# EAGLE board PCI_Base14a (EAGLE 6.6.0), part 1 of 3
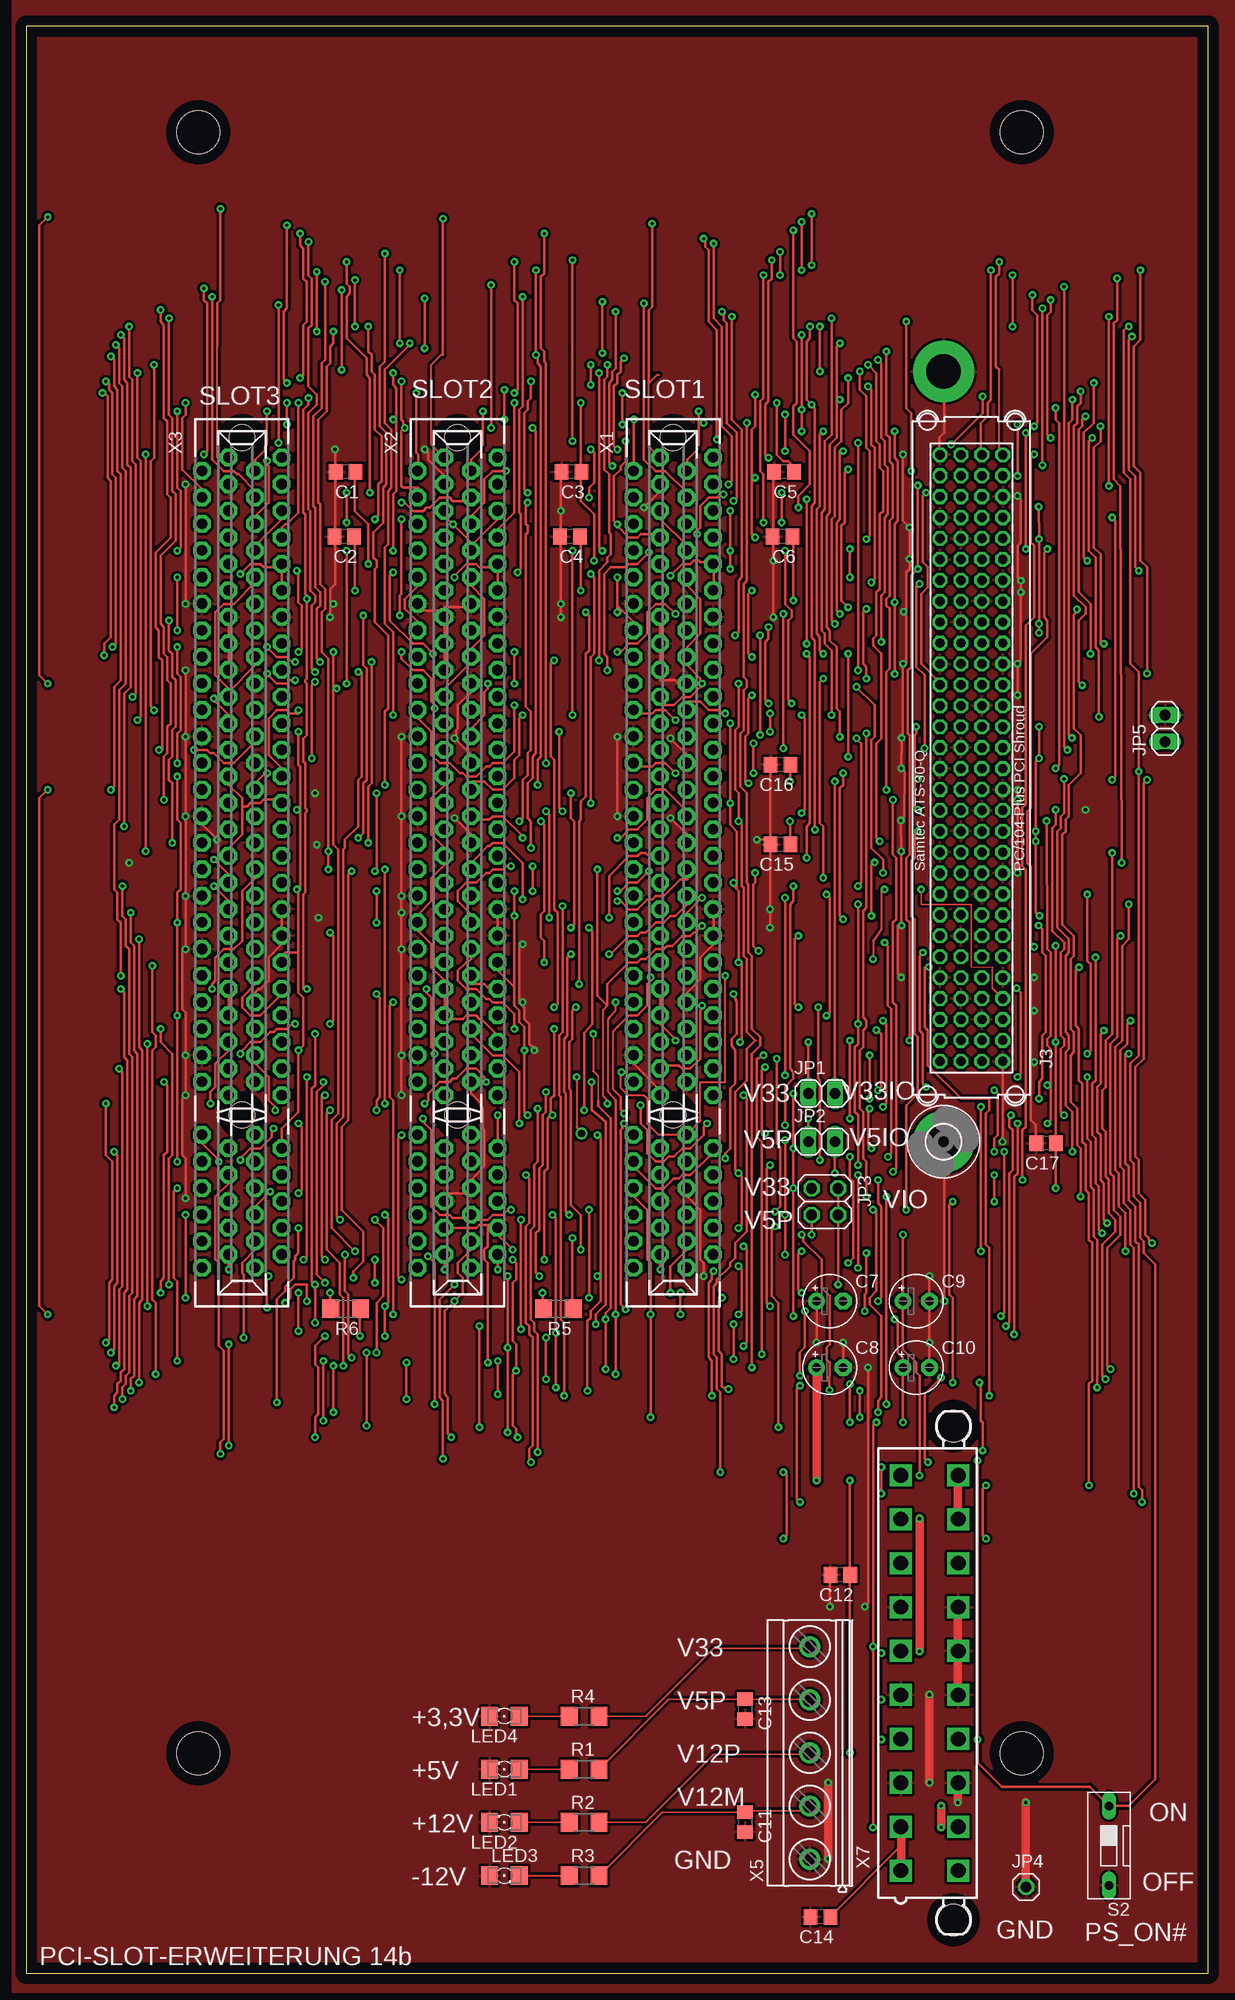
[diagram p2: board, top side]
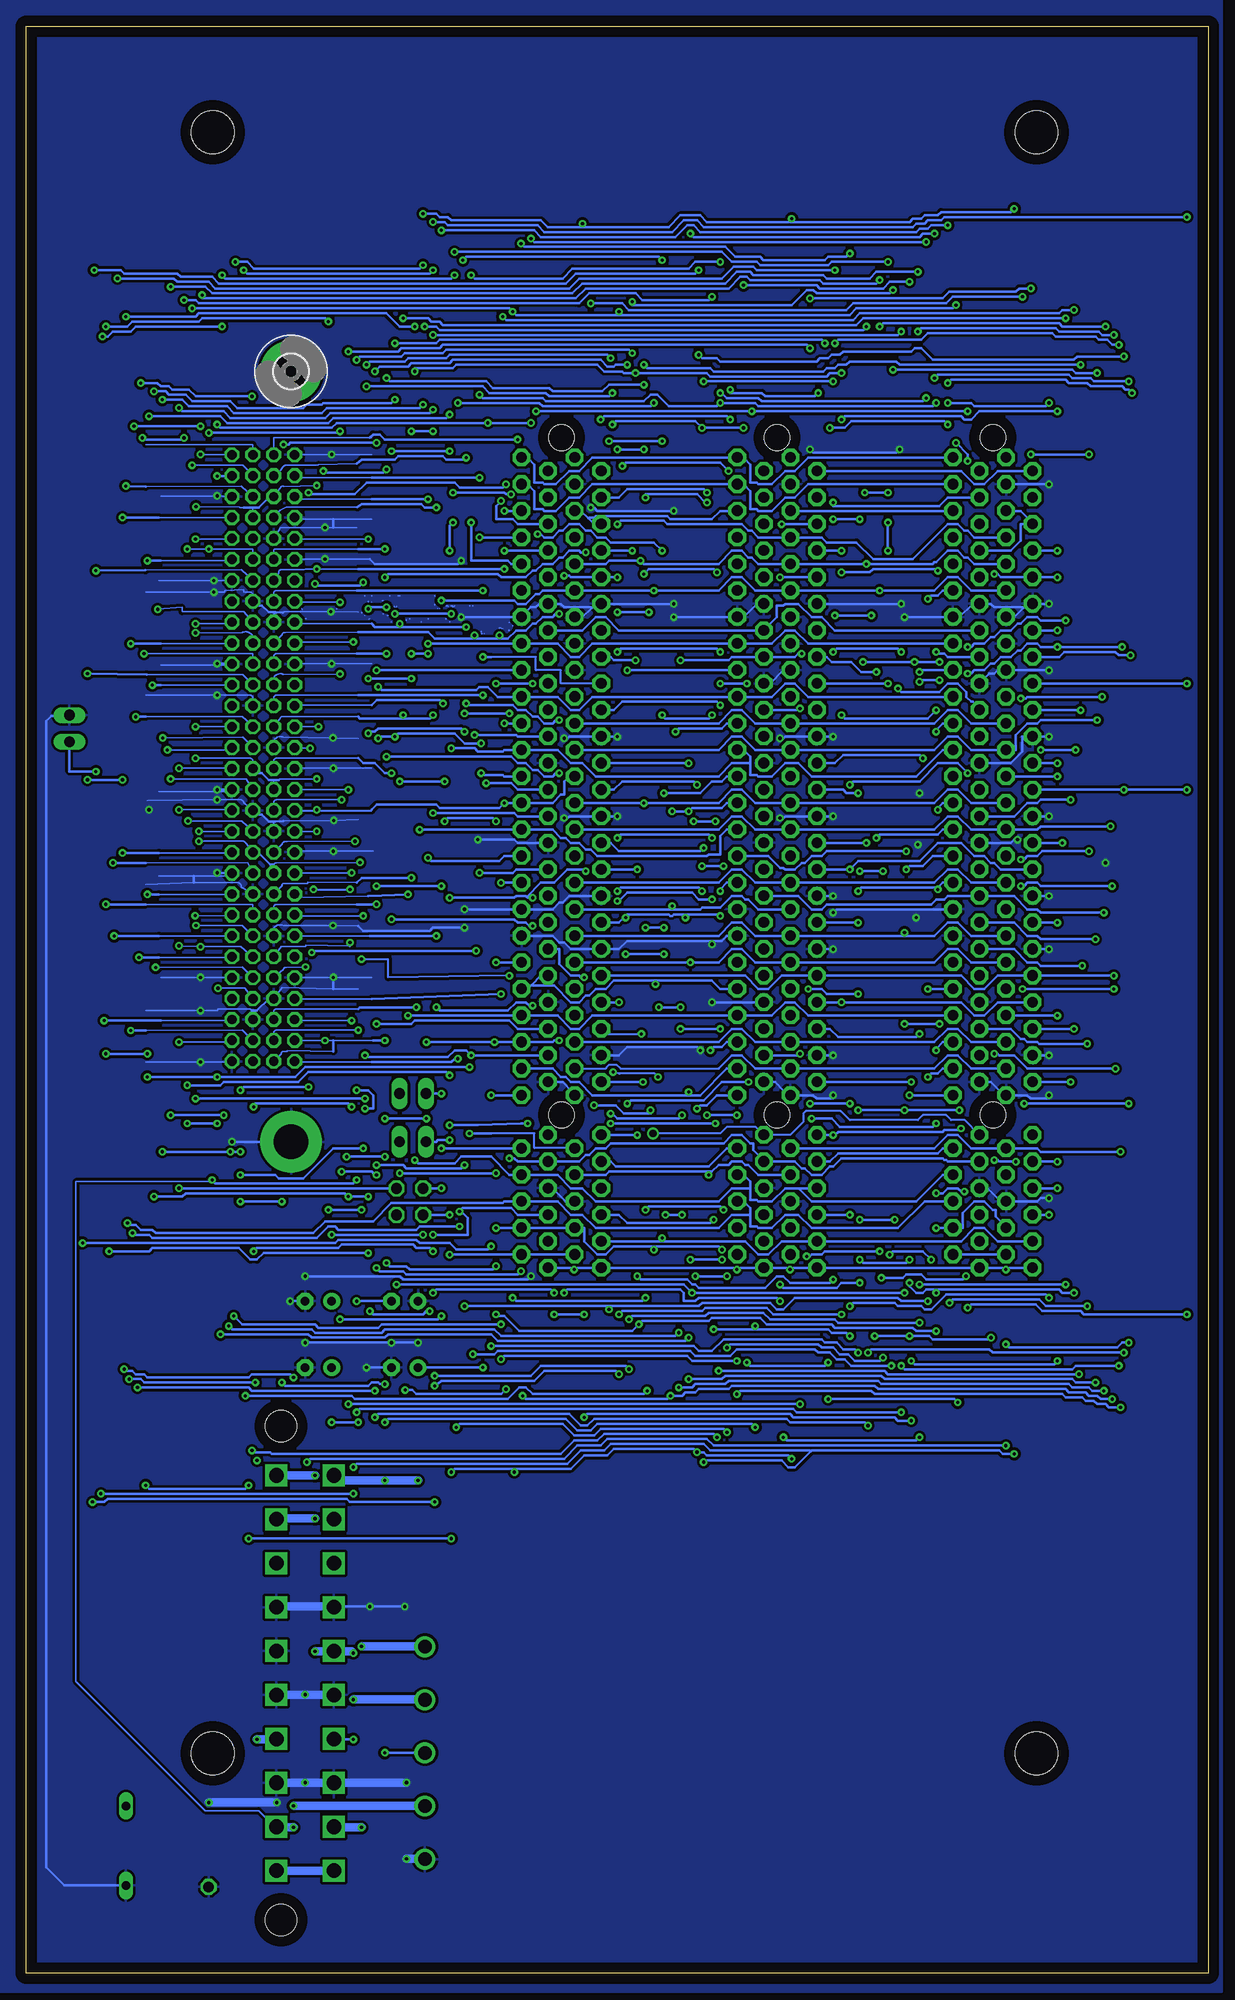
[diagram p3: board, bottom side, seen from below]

Size 113.03 x 186.2 mm. Coordinates in mm from the lower left corner, seen from the top.
Outline: 0,0 113.03,0 113.03,186.2 0,186.2 0,0
Copper layers (1*16): Top 0.035mm / dielectric 1.5mm / Bottom 0.035mm
Design rules "default *": minimum track width 6mil, minimum drill 12mil, track to track 8mil, track to pad 8mil, pad to pad 8mil, via to via 8mil, smd to smd 8mil, copper to edge 40mil, drill to drill 8mil, minimum pad ring 10mil, minimum via ring 8mil, stop-mask expansion 4mil, vias tented up to drill 0mil, thermal gap 10mil
Net classes: 0 signal: width 0.305 mm; 1 supply: width 0.305 mm
Holes 4.1 mm at 16.44,176.05 95.18,176.05 95.18,21.05 16.44,21.05

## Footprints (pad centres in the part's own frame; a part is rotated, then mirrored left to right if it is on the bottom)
C0805 = smd 1.3 x 1.5: 1 -0.95,0; 2 0.95,0
E2,5-5 = drill 0.813 pad 1.6: + -1.27,0 | drill 0.813 pad 1.6 octagon: - 1.27,0
3,3-PAD = drill 3.3 pad 5.842: B3,3 0,0
1X02 = drill 1.016 long: 1 -1.27,0; 2 1.27,0
2X02 = drill 1.016 octagon: 1 -1.27,-1.27; 2 -1.27,1.27; 3 1.27,-1.27; 4 1.27,1.27
1X01 = drill 1.016 octagon: 1 0,0
1206 = smd 1.6 x 1.803: A -1.422,0; C 1.422,0
R1206 = smd 1.6 x 1.803: 1 -1.422,0; 2 1.422,0
DS-01 = drill 0.813 long: 1 0,-3.81; 2 0,3.81
CON-PCI = drill 1.016 pad 1.676 octagon: A1 -38.735,3.81; A2 -37.465,1.27; A3 -36.195,3.81; A4 -34.925,1.27; A5 -33.655,3.81; A6 -32.385,1.27; A7 -31.115,3.81; A8 -29.845,1.27; A9 -28.575,3.81; A10 -27.305,1.27; A11 -26.035,3.81; A12 -24.765,1.27; A13 -23.495,3.81; A14 -22.225,1.27; A15 -20.955,3.81; A16 -19.685,1.27; A17 -18.415,3.81; A18 -17.145,1.27; A19 -15.875,3.81; A20 -14.605,1.27; A21 -13.335,3.81; A22 -12.065,1.27; A23 -10.795,3.81; A24 -9.525,1.27; A25 -8.255,3.81; A26 -6.985,1.27; A27 -5.715,3.81; A28 -4.445,1.27; A29 -3.175,3.81; A30 -1.905,1.27; A31 -0.635,3.81; A32 0.635,1.27; A33 1.905,3.81; A34 3.175,1.27; A35 4.445,3.81; A36 5.715,1.27; A37 6.985,3.81; A38 8.255,1.27; A39 9.525,3.81; A40 10.795,1.27; A41 12.065,3.81; A42 13.335,1.27; A43 14.605,3.81; A44 15.875,1.27; A45 17.145,3.81; A46 18.415,1.27; A47 19.685,3.81; A48 20.955,1.27; A49 22.225,3.81; A52 26.035,1.27; A53 27.305,3.81; A54 28.575,1.27; A55 29.845,3.81; A56 31.115,1.27; A57 32.385,3.81; A58 33.655,1.27; A59 34.925,3.81; A60 36.195,1.27; A61 37.465,3.81; A62 38.735,1.27; B1 -38.735,-1.27; B2 -37.465,-3.81; B3 -36.195,-1.27; B4 -34.925,-3.81; B5 -33.655,-1.27; B6 -32.385,-3.81; B7 -31.115,-1.27; B8 -29.845,-3.81; B9 -28.575,-1.27; B10 -27.305,-3.81; B11 -26.035,-1.27; B12 -24.765,-3.81; B13 -23.495,-1.27; B14 -22.225,-3.81; B15 -20.955,-1.27; B16 -19.685,-3.81; B17 -18.415,-1.27; B18 -17.145,-3.81; B19 -15.875,-1.27; B20 -14.605,-3.81; B21 -13.335,-1.27; B22 -12.065,-3.81; B23 -10.795,-1.27; B24 -9.525,-3.81; B25 -8.255,-1.27; B26 -6.985,-3.81; B27 -5.715,-1.27; B28 -4.445,-3.81; B29 -3.175,-1.27; B30 -1.905,-3.81; B31 -0.635,-1.27; B32 0.635,-3.81; B33 1.905,-1.27; B34 3.175,-3.81; B35 4.445,-1.27; B36 5.715,-3.81; B37 6.985,-1.27; B38 8.255,-3.81; B39 9.525,-1.27; B40 10.795,-3.81; B41 12.065,-1.27; B42 13.335,-3.81; B43 14.605,-1.27; B44 15.875,-3.81; B45 17.145,-1.27; B46 18.415,-3.81; B47 19.685,-1.27; B48 20.955,-3.81; B49 22.225,-1.27; B52 26.035,-3.81; B53 27.305,-1.27; B54 28.575,-3.81; B55 29.845,-1.27; B56 31.115,-3.81; B57 32.385,-1.27; B58 33.655,-3.81; B59 34.925,-1.27; B60 36.195,-3.81; B61 37.465,-1.27; B62 38.735,-3.81 | hole 2.438: 24.13,0; -40.64,0
MKDSN1,5/5-5,08 = drill 1.3 pad 2: 1 -10.181,0.025; 2 -5.101,0.025; 3 -0.021,0.025; 4 5.059,0.025; 5 10.139,0.025
PC104-PLUS = drill 0.9 octagon: J3-A1 -2.825,28.575; J3-A2 -2.825,26.575; J3-A3 -2.825,24.575; J3-A4 -2.825,22.575; J3-A5 -2.825,20.575; J3-A6 -2.825,18.575; J3-A7 -2.825,16.575; J3-A8 -2.825,14.575; J3-A9 -2.825,12.575; J3-A10 -2.825,10.575; J3-A11 -2.825,8.575; J3-A12 -2.825,6.575; J3-A13 -2.825,4.575; J3-A14 -2.825,2.575; J3-A15 -2.825,0.575; J3-A16 -2.825,-1.425; J3-A17 -2.825,-3.425; J3-A18 -2.825,-5.425; J3-A19 -2.825,-7.425; J3-A20 -2.825,-9.425; J3-A21 -2.825,-11.425; J3-A22 -2.825,-13.425; J3-A23 -2.825,-15.425; J3-A24 -2.825,-17.425; J3-A25 -2.825,-19.425; J3-A26 -2.825,-21.425; J3-A27 -2.825,-23.425; J3-A28 -2.825,-25.425; J3-A29 -2.825,-27.425; J3-A30 -2.825,-29.425; J3-B1 -0.825,28.575; J3-B2 -0.825,26.575; J3-B3 -0.825,24.575; J3-B4 -0.825,22.575; J3-B5 -0.825,20.575; J3-B6 -0.825,18.575; J3-B7 -0.825,16.575; J3-B8 -0.825,14.575; J3-B9 -0.825,12.575; J3-B10 -0.825,10.575; J3-B11 -0.825,8.575; J3-B12 -0.825,6.575; J3-B13 -0.825,4.575; J3-B14 -0.825,2.575; J3-B15 -0.825,0.575; J3-B16 -0.825,-1.425; J3-B17 -0.825,-3.425; J3-B18 -0.825,-5.425; J3-B19 -0.825,-7.425; J3-B20 -0.825,-9.425; J3-B21 -0.825,-11.425; J3-B22 -0.825,-13.425; J3-B23 -0.825,-15.425; J3-B24 -0.825,-17.425; J3-B25 -0.825,-19.425; J3-B26 -0.825,-21.425; J3-B27 -0.825,-23.425; J3-B28 -0.825,-25.425; J3-B29 -0.825,-27.425; J3-B30 -0.825,-29.425; J3-C1 1.175,28.575; J3-C2 1.175,26.575; J3-C3 1.175,24.575; J3-C4 1.175,22.575; J3-C5 1.175,20.575; J3-C6 1.175,18.575; J3-C7 1.175,16.575; J3-C8 1.175,14.575; J3-C9 1.175,12.575; J3-C10 1.175,10.575; J3-C11 1.175,8.575; J3-C12 1.175,6.575; J3-C13 1.175,4.575; J3-C14 1.175,2.575; J3-C15 1.175,0.575; J3-C16 1.175,-1.425; J3-C17 1.175,-3.425; J3-C18 1.175,-5.425; J3-C19 1.175,-7.425; J3-C20 1.175,-9.425; J3-C21 1.175,-11.425; J3-C22 1.175,-13.425; J3-C23 1.175,-15.425; J3-C24 1.175,-17.425; J3-C25 1.175,-19.425; J3-C26 1.175,-21.425; J3-C27 1.175,-23.425; J3-C28 1.175,-25.425; J3-C29 1.175,-27.425; J3-C30 1.175,-29.425; J3-D1 3.175,28.575; J3-D2 3.175,26.575; J3-D3 3.175,24.575; J3-D4 3.175,22.575; J3-D5 3.175,20.575; J3-D6 3.175,18.575; J3-D7 3.175,16.575; J3-D8 3.175,14.575; J3-D9 3.175,12.575; J3-D10 3.175,10.575; J3-D11 3.175,8.575; J3-D12 3.175,6.575; J3-D13 3.175,4.575; J3-D14 3.175,2.575; J3-D15 3.175,0.575; J3-D16 3.175,-1.425; J3-D17 3.175,-3.425; J3-D18 3.175,-5.425; J3-D19 3.175,-7.425; J3-D20 3.175,-9.425; J3-D21 3.175,-11.425; J3-D22 3.175,-13.425; J3-D23 3.175,-15.425; J3-D24 3.175,-17.425; J3-D25 3.175,-19.425; J3-D26 3.175,-21.425; J3-D27 3.175,-23.425; J3-D28 3.175,-25.425; J3-D29 3.175,-27.425; J3-D30 3.175,-29.425
5566-20 = drill 1.4 square: 1 18.9,-2.75; 2 14.7,-2.75; 3 10.5,-2.75; 4 6.3,-2.75; 5 2.1,-2.75; 6 -2.1,-2.75; 7 -6.3,-2.75; 8 -10.5,-2.75; 9 -14.7,-2.75; 10 -18.9,-2.75; 11 18.9,2.75; 12 14.7,2.75; 13 10.5,2.75; 14 6.3,2.75; 15 2.1,2.75; 16 -2.1,2.75; 17 -6.3,2.75; 18 -10.5,2.75; 19 -14.7,2.75; 20 -18.9,2.75 | hole 3: 23.6,2.29; -23.6,2.29

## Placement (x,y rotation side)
C1  10n  [C0805]  30.55,143.57 180 top
C2  10n  [C0805]  30.41,137.39 180 top
C3  10n  [C0805]  52.14,143.57 180 top
C4  10n  [C0805]  52,137.39 180 top
C5  10n  [C0805]  72.46,143.57 180 top
C6  10n  [C0805]  72.32,137.39 180 top
C7  47u  [E2,5-5]  76.83,64.28 0 top
C8  47u  [E2,5-5]  76.83,57.93 0 top
C9  47u  [E2,5-5]  85.09,64.28 0 top
C10  47u  [E2,5-5]  85.09,57.93 0 top
C11  100n  [C0805]  68.72,14.48 270 top
C12  100n  [C0805]  77.83,38.1 180 top
C13  100n  [C0805]  68.72,25.27 270 top
C14  100n  [C0805]  75.93,5.4 180 top
C15  100n  [C0805]  72.12,107.95 180 top
C16  100n  [C0805]  72.12,115.57 180 top
C17  100n  [C0805]  97.52,79.38 180 top
H1  MOUNT-PAD-ROUND3.3  [3,3-PAD]  87.71,153.18 0 bottom
H2  MOUNT-PAD-ROUND3.3  [3,3-PAD]  87.71,79.52 0 top
JP1  [1X02]  76.06,84.14 0 top
JP2  [1X02]  76.06,79.54 0 top
JP3  [2X02]  76.36,73.79 270 top
JP4  [1X01]  95.59,8.26 0 top
JP5  [1X02]  108.89,119.05 90 top
LED1  gr  [1206]  45.72,19.52 180 top
LED2  rt  [1206]  45.72,14.44 180 top
LED3  bl  [1206]  45.72,9.35 0 top
LED4  ge  [1206]  45.72,24.6 180 top
R1  220R  [R1206]  53.34,19.51 0 top
R2  1K2  [R1206]  53.34,14.43 0 top
R3  1K5  [R1206]  53.34,9.35 0 top
R4  150R  [R1206]  53.34,24.59 0 top
R5  4K7  [R1206]  50.87,63.56 180 top
R6  4K7  [R1206]  30.55,63.56 180 top
S2  [DS-01]  103.51,12.21 180 top
X1  [CON-PCI]  61.86,106.21 270 top
X2  [CON-PCI]  41.24,106.21 270 top
X3  [CON-PCI]  20.62,106.21 270 top
X5  MKDSN1,5/5-5,08  [MKDSN1,5/5-5,08]  74.93,21.1 90 top
X6  PC104_USB_SUBD  [PC104-PLUS]  90.53,115.78 180 top
X7  5566-20  [5566-20]  86.36,28.72 270 top

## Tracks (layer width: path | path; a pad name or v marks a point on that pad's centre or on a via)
ACK64#  (via drill 0.3)
  Top 0.254: v52.23,70.31 52.23,63.65 R5.1
  Bottom 0.254: X3.B60 16.83,70 20.16,70 21.43,71.27 22.38,71.27 23.65,70 37.31,70 X2.B60 37.46,70 40.8,70 42.07,68.73 43.02,68.73 44.29,70 52.23,70 | 52.23,70 57.94,70 X1.B60 | 52.23,70 v52.23,70.31
AD00  (via drill 0.3)
  Top 0.254: v71.6,72.85 72.07,73.33 72.07,79.05 71.75,79.36 v71.75,87.46 | v37.94,81.74 38.1,81.59 38.1,81.27 38.73,80.63 38.73,73.33 39.53,72.54 40.48,72.54 40.8,72.22 42.07,72.22 42.39,72.54 X2.A58 42.54,72.54 42.54,72.06 44.13,72.06 44.61,72.54 45.56,72.54 46.04,73.01 v46.35,73.01 | v26.03,81.27 26.35,80.95 26.35,74.92 v26.03,74.6 | v23.34,74.76 21.91,73.33 21.91,72.7 X3.A58 | v74.14,70.63 74.29,70.47 74.29,70 76.04,68.25 76.04,65.55 76.83,64.76 76.83,60.15 76.52,59.84 76.52,58.73 76.83,58.41 v76.79,55.79 | v67.15,55.87 66.83,55.87 66.52,56.19 66.52,59.2 66.2,59.52 66.2,64.28 v66.52,64.6 | v53.82,73.01 v53.82,64.6
  Bottom 0.152: X6.J3-D1 87.36,87.14 80.01,87.14
  Bottom 0.254: v71.75,87.46 72.07,87.46 72.39,87.14 80.01,87.14 | X1.A58 63.18,72.54 66.04,72.54 66.67,73.17 71.28,73.17 v71.6,72.85 71.44,72.85 70.8,72.22 70.8,70.63 v74.14,70.63 | v37.94,81.74 36.04,81.74 35.24,80.95 26.35,80.95 v26.03,81.27 | v26.03,74.6 25.4,74.6 24.92,75.08 23.97,75.08 23.65,74.76 v23.34,74.76 | v76.79,55.79 76.12,55.79 75.72,55.39 67.63,55.39 v67.15,55.87 | v66.52,64.6 66.2,64.28 54.13,64.28 v53.82,64.6 | v53.82,73.01 53.5,73.33 46.67,73.33 v46.35,73.01
AD01  (via drill 0.3)
  Top 0.254: v15.24,64.6 v15.24,72.54 | v34.29,72.54 34.61,72.22 34.61,64.12 v34.29,63.81 v34.29,60.95 | v47.31,61.58 v47.31,72.06 | v81.28,90.2 81.76,89.84 81.76,84.76 v81.44,84.44 | v80.64,82.7 80.49,82.54 80.49,79.2 v80.8,78.89 | v92.55,73.81 v92.55,76.35 | v88.58,73.81 88.26,73.49 88.26,64.92 88.58,64.6 v88.58,56.5 | v78.74,52.69 v78.74,56.34 | v43.34,61.9 v43.34,52.22
  Bottom 0.152: X6.J3-C2 89.36,89.9 arc90 89.11,90.2 v81.28,90.2 81.28,90.16
  Bottom 0.254: v15.24,72.54 16.67,72.54 X3.B58 | v15.24,64.6 15.56,64.92 25.08,64.92 26.51,63.49 27.15,63.49 27.46,63.81 29.69,63.81 30,64.12 33.97,64.12 v34.29,63.81 | v34.29,72.54 37.31,72.54 X2.B58 | v47.31,72.06 47.62,71.74 55.56,71.74 56.36,72.54 57.94,72.54 X1.B58 | 43.34,61.58 36.35,61.58 36.04,61.27 34.61,61.27 v34.29,60.95 | 43.34,61.58 v47.31,61.58 | v81.44,84.44 80.33,84.44 79.85,83.97 79.85,82.7 v80.64,82.7 | v80.8,78.89 83.66,78.89 86.52,76.03 88.9,76.03 89.22,76.35 v92.55,76.35 | v88.58,73.81 v92.55,73.81 | v88.58,56.5 88.26,56.19 80.33,56.19 80.01,56.5 79.37,56.5 79.22,56.34 v78.74,56.34 | v78.74,52.69 78.42,53.01 61.44,53.01 60.32,51.9 59.05,51.9 58.42,52.53 43.66,52.53 v43.34,52.22 | 43.34,61.58 v43.34,61.9
AD02  (via drill 0.3)
  Top 0.254: v103.03,90.16 102.71,89.84 102.71,85.08 102.39,84.76 102.39,80.47 102.71,80.16 102.71,75.87 103.03,75.55 103.03,72.06 v103.35,71.74
  Bottom 0.152: X6.J3-B2 92.39,90.2 101.6,90.16
  Bottom 0.254: 43.81,72.54 43.81,71.43 43.18,71.43 43.02,71.27 41.75,71.27 40.48,72.54 39.21,72.54 37.94,71.27 29.69,71.27 27.15,73.81 24.45,73.81 X3.A57 | 43.81,72.54 43.81,73.17 44.45,73.81 44.93,73.81 X2.A57 | 43.81,72.54 45.56,72.54 46.83,71.27 58.58,71.27 59.85,72.54 60.96,72.54 62.23,73.81 65.56,73.81 X1.A57 65.72,73.81 67.31,73.81 67.47,73.65 78.1,73.65 79.85,71.9 84.45,71.9 85.57,70.79 100.65,70.79 100.96,71.11 102.08,71.11 102.55,71.58 103.19,71.58 v103.35,71.74 | v103.03,90.16 101.6,90.16
AD03  (via drill 0.3)
  Top 0.254: v14.45,75.08 14.13,74.76 14.13,66.5 14.45,66.19 v14.45,58.57 | v28.42,52.85 v28.42,58.57 | v59.69,53.17 v59.69,63.01 59.69,67.93 59.37,68.25 59.37,73.01 58.1,74.28 58.1,75.08 X1.B56 | v81.91,91.11 82.23,90.79 82.23,83.17 v81.91,82.86 | v91.28,69.04 v91.28,82.86 | v74.14,69.04 73.82,68.73 73.82,65.39 v74.14,65.08 | v62.55,63.01 v62.55,65.08
  Bottom 0.152: X6.J3-D3 87.36,91.11 v81.91,91.11
  Bottom 0.254: v14.45,75.08 16.67,75.08 X3.B56 | v14.45,58.57 14.76,58.25 28.1,58.25 v28.42,58.57 | v28.42,52.85 29.69,52.85 30,53.17 39.69,53.17 40,53.49 59.37,53.49 v59.69,53.17 | v81.91,82.86 82.23,83.17 91.12,83.17 91.28,83.01 v91.28,82.86 | v91.28,69.04 90.96,69.36 83.18,69.36 82.87,69.68 76.04,69.68 75.72,69.36 74.45,69.36 v74.14,69.04 | v74.14,65.08 73.82,65.39 62.86,65.39 v62.55,65.08 | v59.69,63.01 v62.55,63.01
AD04  (via drill 0.3)
  Top 0.254: v75.72,92.38 75.72,85.55 75.88,85.4 v75.88,77.78
  Bottom 0.152: X6.J3-C3 89.36,91.97 arc90 89.11,92.22 81.28,92.22
  Bottom 0.254: 43.81,75.08 43.81,73.97 43.18,73.97 43.02,73.81 41.75,73.81 40.48,75.08 39.21,75.08 39.13,75 | 43.81,75.08 43.81,75.71 44.45,76.35 44.93,76.35 X2.A55 | 39.13,75 37.94,73.81 27.94,73.81 25.4,76.35 24.45,76.35 X3.A55 | 43.81,75.08 45.56,75.08 46.83,73.81 58.58,73.81 59.85,75.08 60.96,75.08 62.23,76.35 65.56,76.35 X1.A55 65.72,76.35 66.83,76.35 68.58,78.09 71.44,78.09 72.07,77.46 75.56,77.46 v75.88,77.78 | X2.B56 37.46,75.08 39.05,75.08 39.13,75 | 81.28,92.22 81.12,92.38 v75.72,92.38
AD05  (via drill 0.3)
  Top 0.254: v18.57,49.68 18.57,50.79 18.89,51.11 18.89,59.52 18.41,60 18.41,67.93 18.1,68.25 18.1,74.28 19.37,75.55 19.37,76.35 X3.B55 | v48.26,48.88 48.1,49.04 48.1,50.15 48.42,50.47 48.42,60.79 48.1,61.11 48.1,61.9 47.78,62.22 47.78,71.43 48.1,71.74 48.1,76.03 v47.78,76.35 | v105.57,91.11 105.25,90.79 105.25,88.89 104.62,88.25 104.62,77.14 104.93,76.82 104.93,73.65 105.57,73.01 105.57,69.68 105.89,69.36 v105.89,45.87 | v81.76,48.41 v81.76,45.87
  Bottom 0.152: X6.J3-A3 arc90 93.46,91.11 100.17,91.11
  Bottom 0.254: v18.57,49.68 19.68,49.68 20,49.99 37.94,49.99 38.02,49.91 | 38.02,49.91 39.53,48.41 40.16,48.41 40.8,49.04 48.1,49.04 v48.26,48.88 | X1.B55 60.48,76.35 57.63,76.35 57.31,76.66 48.1,76.66 v47.78,76.35 47.94,76.66 47.47,76.66 46.83,77.3 45.88,77.3 45.56,77.62 44.61,77.62 44.29,77.3 43.97,77.3 43.02,76.35 40,76.35 X2.B55 | v105.57,91.11 100.17,91.11 | v81.76,45.87 v105.89,45.87 | v81.76,48.41 81.44,48.72 61.28,48.72 60.01,49.99 57.78,49.99 57.15,50.63 48.26,50.63 47.62,49.99 38.1,49.99 38.02,49.91
AD06  (via drill 0.3)
  Top 0.254: v67.63,93.65 67.94,92.86 67.94,89.84 67.47,89.36 67.47,88.73 67.79,88.25 67.79,85.08 67.31,84.6 67.31,78.89 66.83,78.41 v66.83,77.93
  Bottom 0.152: X6.J3-D4 87.36,93.17 80.01,93.17
  Bottom 0.254: X3.A54 21.91,77.62 24.92,77.62 25.08,77.78 25.24,77.78 25.4,77.93 35.08,77.93 35.88,77.14 36.19,77.14 36.99,76.35 37.94,76.35 38.58,76.98 38.89,76.98 39.53,77.62 42.39,77.62 X2.A54 42.54,77.78 43.5,78.73 43.5,79.36 43.81,79.36 44.61,80.16 45.56,80.16 46.35,79.36 57.15,79.36 57.63,78.89 58.58,78.89 59.21,78.25 59.53,78.25 60.17,77.62 63.02,77.62 X1.A54 63.18,77.62 66.04,77.62 66.36,77.93 v66.83,77.93 | v67.63,93.65 80.01,93.17
AD07  (via drill 0.3)
  Top 0.254: v70.64,80.32 70.33,80.63 70.33,86.35 v70.64,86.67 | v94.77,85.71 95.09,86.03 95.09,93.81 v94.69,94.21 | v8.41,78.57 8.73,78.25 8.73,66.03 8.41,65.71 8.41,59.68 v8.1,59.36 | v32.54,52.38 v32.54,59.36 | v79.69,55.71 v79.69,53.17 | v102.39,56.03 102.39,70.16 102.08,70.47 102.08,74.92 101.76,75.24 101.76,79.52 101.44,79.84 v101.44,85.71
  Bottom 0.152: X6.J3-B4 92.15,94.21 v94.69,94.21
  Bottom 0.203: X1.B53 64.45,78.91 64.45,80.32 68.58,80.32
  Bottom 0.254: X2.B53 39.85,78.89 26.19,78.89 24.92,80.16 23.97,80.16 22.7,78.89 19.37,78.89 X3.B53 19.21,78.89 16.35,78.89 16.03,78.57 v8.41,78.57 | v70.64,80.32 68.58,80.32 | v70.64,86.67 86.36,86.67 87.31,85.71 v94.77,85.71 v101.44,85.71 | v8.1,59.36 20.64,59.36 20.95,59.68 32.23,59.68 v32.54,59.36 | v32.54,52.38 32.86,52.69 40,52.69 40.32,53.01 58.74,53.01 59.37,52.38 60.01,52.38 61.12,53.49 79.37,53.49 v79.69,53.17 | v79.69,55.71 91.44,55.71 91.76,56.03 v102.39,56.03
AD08  (via drill 0.3)
  Top 0.254: v18.41,77.62 18.41,77.78 16.83,79.36 16.83,80.16 X3.B52 | v20.48,77.78 20.64,77.93 20.64,78.09 21.43,78.89 22.38,78.89 23.49,80 23.49,80.63 v23.65,80.79 | v54.61,80.16 54.93,79.84 54.93,66.98 v54.61,66.66 54.93,66.82 54.93,64.28 53.97,63.33 53.97,62.69 53.66,62.38 v53.66,55.71 | v35.88,66.35 35.56,66.66 35.56,79.84 v35.88,80.16 | v86.32,96.23 85.88,96.19 85.88,90.48 86.2,90.16 86.2,86.82 89.38,83.65 92.07,83.65 92.07,82.54 91.76,82.22 91.76,69.68 92.07,69.36 v92.07,55.23
  Bottom 0.152: X6.J3-C5 88.45,95.98 arc90 88.15,96.19 v86.32,96.23
  Bottom 0.254: v18.41,77.62 20,77.62 20.16,77.78 v20.48,77.78 | v23.65,80.79 23.81,80.63 25.24,80.63 25.4,80.47 35.4,80.47 35.72,80.16 v35.88,80.16 37.31,80.16 X2.B52 | v54.61,80.16 57.94,80.16 X1.B52 | v54.61,66.66 54.29,66.35 49.85,66.35 49.37,65.87 49.05,65.87 48.74,65.55 42.39,65.55 41.27,66.66 40.64,66.66 40,66.03 36.19,66.03 v35.88,66.35 | v92.07,55.23 81.91,55.23 81.6,54.92 66.99,54.92 65.88,56.03 65.25,56.03 64.61,55.39 53.97,55.39 v53.66,55.71
AD09  (via drill 0.3)
  Top 0.254: v48.89,82.7 48.89,77.62 48.58,77.3 48.58,71.43 48.26,71.11 48.26,62.54 48.58,62.22 48.58,61.42 48.89,61.11 v48.89,49.84 | v72.39,47.93 72.71,47.61 72.71,41.9 v72.39,41.58 | v91.76,41.58 91.44,41.9 91.44,46.34 v91.76,46.66 | v101.6,46.66 101.6,56.34 101.92,56.66 101.92,69.84 101.6,70.16 101.6,74.6 101.28,74.92 101.28,79.2 100.96,79.52 100.96,85.08 100.65,85.4 100.65,90.32 100.33,90.63 100.33,95.87 v100.65,96.19 | v28.57,83.97 28.26,83.97 28.26,68.57 v28.57,68.25 | v33.34,66.03 v33.34,68.25 | v40.96,65.87 39.53,64.44 39.53,55.07 39.85,54.76 v39.85,49.2 | v68.58,83.97 68.9,83.65 68.9,70.95 67.79,69.84 67.79,68.41 67.31,67.93 67.31,67.62 66.04,66.35 66.04,66.03 65.72,65.71 65.72,59.2 66.04,58.88 66.04,55.87 66.36,55.55 v66.36,47.93
  Bottom 0.152: X6.J3-B5 92.35,96.23 v100.65,96.19
  Bottom 0.254: v48.89,82.7 48.58,83.01 47.94,83.01 46.99,83.97 45.08,83.97 X2.A49 | 66.36,48.25 72.07,48.25 v72.39,47.93 | 66.36,48.25 60.96,48.25 59.69,49.52 57.47,49.52 56.83,50.15 49.21,50.15 v48.89,49.84 48.26,49.84 47.94,49.52 40.16,49.52 v39.85,49.2 | v91.76,41.58 v72.39,41.58 | v91.76,46.66 92.07,46.34 101.28,46.34 v101.6,46.66 | v28.57,83.97 24.45,83.97 X3.A49 | v28.57,68.25 28.89,67.93 33.02,67.93 v33.34,68.25 | v33.34,66.03 35.08,66.03 35.56,65.55 40.64,65.55 v40.96,65.87 | v68.58,83.97 65.72,83.97 X1.A49 | 66.36,48.25 v66.36,47.93
AD10  (via drill 0.3)
  Top 0.254: v13.18,85.24 13.49,84.92 13.49,78.57 13.18,78.25 13.18,66.5 12.86,66.19 v12.86,65.08 | v28.57,66.03 27.78,66.82 27.78,84.28 28.42,84.92 v28.42,85.24 | v54.05,85.24 54.05,82.54 55.4,81.43 55.4,63.96 54.45,63.01 v54.45,62.06 | v26.03,65.08 v26.03,61.42 | v82.07,98.57 82.39,98.25 82.39,92.54 82.71,92.22 82.71,78.41 v82.39,78.09 | v78.74,78.09 78.74,76.03 79.06,75.71 79.06,68.41 v78.58,67.93 | v68.1,67.62 68.42,67.3 68.42,63.33 v68.1,63.01
  Bottom 0.152: X6.J3-C6 88.65,98.21 86.32,98.21 86.32,98.33 82.07,98.25
  Bottom 0.254: v13.18,85.24 16.67,85.24 X3.B48 | v12.86,65.08 13.97,65.08 14.29,65.39 26.03,65.39 | 26.03,65.39 26.99,65.39 27.3,65.08 27.94,65.08 28.57,65.71 v28.57,66.03 | v28.42,85.24 37.31,85.24 X2.B48 | v54.05,85.24 57.94,85.24 X1.B48 | v26.03,61.42 27.94,61.42 28.26,61.74 35.72,61.74 36.04,62.06 42.23,62.06 42.86,62.69 47.47,62.69 47.78,62.38 54.13,62.38 v54.45,62.06 55.09,61.42 65.88,61.42 67.31,62.85 67.94,62.85 v68.1,63.01 | 26.03,65.39 v26.03,65.08 | v82.07,98.57 82.07,98.25 | v78.74,78.09 v82.39,78.09 | v78.58,67.93 78.26,67.62 76.68,67.62 76.36,67.3 68.42,67.3 v68.1,67.62
AD11  (via drill 0.3)
  Top 0.254: v26.83,85.71 26.83,68.57 v26.51,68.25 | v30.48,68.73 30.48,65.23 30.8,64.92 30.8,59.2 v31.11,58.88 | v46.04,66.66 v46.04,59.84 v46.04,51.74 | v49.05,66.66 48.74,66.98 48.74,70.79 49.05,71.11 49.05,76.98 49.37,77.3 49.37,82.06 49.69,82.38 v49.69,84.28 | v102.23,97.14 102.23,85.4 101.92,85.08 101.92,80.16 102.23,79.84 102.23,75.55 102.55,75.24 102.55,71.11 v102.87,70.79 | v71.6,71.43 71.28,71.11 71.28,64.76 71.91,64.12 v71.91,52.22
  Bottom 0.152: X6.J3-A6 arc90 93.43,97.14 100.33,97.14
  Bottom 0.254: 49.69,83.97 58.9,83.97 60.17,85.24 60.96,85.24 61.44,85.71 61.91,85.71 62.71,86.51 65.56,86.51 X1.A47 | 49.69,83.97 48.58,83.97 46.04,86.51 45.08,86.51 X2.A47 | v26.83,85.71 26.51,86.03 25.88,86.03 25.4,86.51 24.45,86.51 X3.A47 | v26.51,68.25 27.3,69.04 30.16,69.04 v30.48,68.73 | v31.11,58.88 31.43,58.57 33.81,58.57 34.45,59.2 35.24,59.2 35.88,59.84 36.99,59.84 37.31,60.15 45.72,60.15 v46.04,59.84 | v49.05,66.66 v46.04,66.66 | 49.69,83.97 v49.69,84.28 | v102.23,97.14 100.33,97.14 | v102.87,70.79 102.71,70.63 101.28,70.63 100.96,70.31 85.25,70.31 84.14,71.43 83.5,71.43 83.18,71.11 75.72,71.11 75.41,71.43 v71.6,71.43 | v71.91,52.22 71.6,52.53 61.75,52.53 60.64,51.42 58.74,51.42 58.1,52.06 46.35,52.06 v46.04,51.74
AD12  (via drill 0.3)
  Top 0.254: v73.82,99.21 73.5,98.89 73.5,92.7 v73.82,92.38 | v64.61,92.54 64.61,92.22 64.45,92.06 64.45,87.46 63.5,86.51 62.71,86.51 62.39,86.82 60.64,86.82 60.64,86.67 X1.B47
  Bottom 0.152: X6.J3-D7 80.17,99.21
  Bottom 0.203: 60.48,86.51 57.63,86.51 57.55,86.59 57.55,86.67 57.31,86.9 56.59,86.9 56.2,86.51 46.83,86.51
  Bottom 0.254: X3.B47 19.37,86.51 22.7,86.51 23.97,87.78 24.92,87.78 26.19,86.51 39.85,86.51 X2.B47 40,86.51 43.34,86.51 44.61,87.78 45.56,87.78 46.83,86.51 | 60.48,86.51 X1.B47 | v73.82,99.21 80.17,99.21 | v73.82,92.38 73.5,92.06 66.99,92.06 66.2,92.86 65.25,92.86 64.93,92.54 v64.61,92.54
AD13  (via drill 0.3)
  Top 0.254: v23.81,82.54 23.81,82.86 23.18,83.49 23.18,85.71 21.91,86.98 21.91,87.78 X3.A46 | v29.05,82.54 28.73,82.22 28.73,69.2 30,67.93 30,64.92 30.32,64.6 v30.32,58.09 | v70.33,59.2 70.33,79.52 69.85,80 69.85,87.46 v70.48,87.78 | v39.05,87.94 39.05,88.25 38.73,88.57 38.73,93.33 38.26,93.81 v38.26,94.13 | v33.5,93.65 33.81,93.33 33.81,83.81 33.5,83.49 v33.5,82.54 | v96.8,100.2 97.15,99.84 97.15,97.62 97.47,97.3 97.47,90 97.15,89.68 97.15,85.55 96.84,85.24 v96.84,83.65 | v80.64,87.78 v80.64,83.65
  Bottom 0.152: X6.J3-B7 92.35,100.2 v96.8,100.2
  Bottom 0.254: v23.81,82.54 v29.05,82.54 v33.5,82.54 | v30.32,58.09 34.13,58.09 34.77,58.73 35.56,58.73 36.19,59.36 37.31,59.36 37.62,59.68 45.08,59.68 45.72,59.04 49.05,59.04 49.53,59.52 67.94,59.52 68.26,59.2 v70.33,59.2 | X1.A46 63.18,87.78 v70.48,87.78 70.96,88.25 72.07,88.25 72.71,87.62 80.49,87.62 v80.64,87.78 | v39.05,87.94 39.21,87.78 42.39,87.78 X2.A46 | v38.26,94.13 36.99,94.13 36.51,93.65 v33.5,93.65 | v80.64,83.65 v96.84,83.65
AD14  (via drill 0.3)
  Top 0.254: v104.62,99.21 104.3,98.89 104.3,89.52 103.66,88.89 103.66,76.51 103.98,76.19 103.98,73.01 104.62,72.38 104.62,70.63 103.35,69.36 103.35,58.09 v103.66,57.77 | v87.47,56.98 85.88,55.39 85.88,49.2 v86.2,48.88 | v19.37,60.15 v19.37,50.47 | v7.62,60.31 7.94,60.63 7.94,66.03 8.25,66.35 8.25,77.62 7.62,78.25 v7.62,83.17 | v17.62,83.17 17.62,84.28 18.1,84.76 18.1,86.98 19.37,88.25 19.37,89.05 X3.B45
  Bottom 0.152: X6.J3-A7 arc90 X6.J3-A7 100.33,99.21
  Bottom 0.254: X3.B45 19.37,89.05 22.7,89.05 23.97,90.32 24.92,90.32 26.19,89.05 39.85,89.05 X2.B45 40,89.05 43.34,89.05 44.61,90.32 45.56,90.32 46.83,89.05 60.48,89.05 X1.B45 | v104.62,99.21 100.33,99.21 | v103.66,57.77 103.5,57.61 102.87,57.61 102.55,57.3 101.76,57.3 101.44,56.98 91.76,56.98 91.44,57.3 87.79,57.3 v87.47,56.98 | v86.2,48.88 85.88,49.2 61.59,49.2 60.32,50.47 58.1,50.47 57.47,51.11 47.94,51.11 47.31,50.47 v19.37,50.47 | v19.37,60.15 19.05,59.84 8.73,59.84 8.25,60.31 v7.62,60.31 | v17.62,83.17 v7.62,83.17
AD15  (via drill 0.3)
  Top 0.254: v11.59,63.81 v11.59,88.89 | v24.76,64.12 25.24,64.6 25.24,65.39 25.72,65.87 26.83,65.87 v26.83,64.28 | v71.12,63.81 70.8,64.12 70.8,76.98 v71.12,77.3 | v79.53,77.3 79.53,82.06 79.22,82.38 79.22,88.57 79.53,88.89 v79.53,90.79 v79.53,102.22 | v47.15,81.27 47.15,86.19 45.56,87.78 44.61,87.78 42.54,89.84 42.54,90.32 X2.A44 | v57.15,81.27 56.99,81.11 56.99,80.79 56.83,80.63 56.83,63.96 v57.31,63.49
  Bottom 0.152: X6.J3-C8 89.36,101.97 arc90 89.11,102.22 81.44,102.22
  Bottom 0.254: v11.59,88.89 16.19,88.89 16.35,89.05 17.3,89.05 17.62,89.36 17.94,89.36 18.89,90.32 21.75,90.32 X3.A44 | v11.59,63.81 15.56,63.81 16.19,64.44 24.45,64.44 v24.76,64.12 | v26.83,64.28 29.37,64.28 29.69,64.6 39.53,64.6 40.64,63.49 41.27,63.49 41.91,64.12 48.42,64.12 48.74,63.81 57.31,63.81 | v71.12,63.81 57.31,63.81 | v71.12,77.3 71.44,76.98 76.68,76.98 76.99,77.3 v79.53,77.3 | 81.44,102.22 v79.53,102.22 | v57.15,81.27 v47.15,81.27 | 57.31,63.81 v57.31,63.49 | v79.53,90.79 76.2,90.79 75.88,91.11 66.83,91.11 66.04,90.32 63.18,90.32 X1.A44
AD16  (via drill 0.3)
  Top 0.254: v47.47,102.7 47.47,106.19 45.56,108.1 44.61,108.1 44.29,107.78 44.13,107.78 42.54,106.19 42.54,105.72 X2.A32 | v56.51,102.54 56.83,102.54 57.63,101.75 58.42,101.75 59.37,102.7 59.85,102.7 60.17,103.02 60.96,103.02 62.55,104.6 63.18,104.6 63.18,105.56 X1.A32 | v17.78,94.13 17.78,94.6 18.1,94.92 18.1,97.14 18.89,97.94 19.84,97.94 20.64,98.73 20.64,103.49 21.91,104.76 21.91,105.56 X3.A32 | v9.05,94.13 9.37,93.81 9.37,87.62 9.68,87.3 9.68,65.39 9.37,65.08 9.37,57.77 9.05,57.46 9.05,56.66 8.73,56.34 8.73,55.55 8.41,55.23 v8.41,54.12 | v45.08,58.57 v45.08,55.39 | v67.63,62.06 v67.63,58.73 | v93.19,62.85 93.5,63.17 v93.5,78.57 | v100.01,78.57 100.01,82.38 99.38,83.01 99.38,88.09 99.69,88.41 99.69,89.68 99.38,90 99.38,97.3 99.69,97.62 99.69,98.89 98.58,100 98.58,109.21 98.9,109.53 98.9,110.64 99.22,110.95 v99.22,114.21 | v69.69,105.24 69.69,104.29 69.53,104.13 69.53,98.25 v70.01,97.78 | v85.72,97.62 85.41,97.3 85.41,90.16 85.72,89.84 85.72,85.08 v86.04,84.76 | v92.55,84.44 92.87,84.13 92.87,80.16 92.55,79.84 v92.55,78.57
  Bottom 0.152: X6.J3-B14 91.99,114.21 v99.22,114.21
  Bottom 0.254: v47.47,102.7 48.74,102.7 49.37,103.33 55.56,103.33 56.36,102.54 v56.51,102.54 | v9.05,94.13 v17.78,94.13 | v8.41,54.12 9.52,54.12 9.84,54.44 10.64,54.44 10.95,54.76 11.75,54.76 12.06,55.07 13.65,55.07 13.97,55.39 31.91,55.39 32.23,55.71 44.77,55.71 v45.08,55.39 | v45.08,58.57 49.37,58.57 49.85,59.04 67.31,59.04 v67.63,58.73 | v67.63,62.06 79.06,62.06 79.37,61.74 85.09,61.74 85.41,62.06 92.39,62.06 v93.19,62.85 | v100.01,78.57 v93.5,78.57 v92.55,78.57 | v69.69,105.24 66.52,105.24 66.2,105.56 63.18,105.56 X1.A32 | v70.01,97.78 85.57,97.78 v85.72,97.62 | v86.04,84.76 92.23,84.76 v92.55,84.44
AD17  (via drill 0.3)
  Top 0.203: v55.56,83.17 55.56,83.49 55.17,83.89 55.17,92.14 55.56,92.54
  Top 0.254: v54.61,105.56 54.61,93.49 55.48,92.62 | 55.56,92.54 55.48,92.62 | v43.97,85.24 43.81,85.4 43.81,85.71 43.02,86.51 42.07,86.51 41.12,85.55 40.8,85.55 40.48,85.24 39.53,85.24 38.42,84.13 38.42,83.49 v38.1,83.17 | v34.29,105.56 v34.29,83.17 | v78.1,114.76 78.1,113.65 77.79,113.34 77.79,101.11 v78.1,100.79 | v64.61,100.16 63.98,99.52 63.82,99.52 63.5,99.21 62.71,99.21 61.75,98.25 61.28,98.25 60.96,97.94 60.17,97.94 59.21,96.98 58.74,96.98 58.42,96.67 57.63,96.67 55.56,94.6 55.56,92.7 55.48,92.62
  Bottom 0.152: X6.J3-C15 89.36,115.94 arc90 89.11,116.19 81.28,116.19
  Bottom 0.254: v54.61,105.56 57.94,105.56 X1.B32 | v55.56,83.17 55.24,83.49 48.26,83.49 46.51,85.24 v43.97,85.24 | v34.29,83.17 v38.1,83.17 | X2.B32 37.31,105.56 v34.29,105.56 33.5,106.35 27.62,106.35 25.88,108.1 23.65,108.1 22.38,106.83 21.43,106.83 20.8,106.19 20.48,106.19 19.84,105.56 16.83,105.56 X3.B32 | 81.28,116.19 80.8,115.72 79.69,115.72 78.74,114.76 v78.1,114.76 | v78.1,100.79 66.36,100.79 66.04,100.48 65.25,100.48 64.93,100.16 v64.61,100.16
AD18  (via drill 0.3)
  Top 0.254: v28.89,105.56 v28.89,107.3 28.89,125.72 28.26,126.35 28.26,130.16 28.57,130.48 28.57,132.39 28.1,132.86 28.1,140.48 27.94,140.64 27.94,148.58 28.73,149.37 28.73,153.66 29.05,153.98 29.05,155.56 29.37,155.88 v29.37,156.99 | v74.14,156.67 v74.14,149.53 v74.14,147.47 | v98.42,149.69 98.42,148.58 98.74,148.26 98.74,115.56 v98.42,115.24 | v74.61,106.67 74.61,109.68 74.93,110 74.93,125.88 v74.61,126.19 | v76.2,126.19 75.88,126.51 75.88,127.78 75.56,128.1 75.56,140.01 75.88,140.32 75.88,147.15 v76.2,147.47
  Bottom 0.152: X6.J3-A15 arc-90 93.39,115.24 v98.42,115.24
  Bottom 0.254: v28.89,105.56 28.57,105.87 27.3,105.87 26.35,106.83 24.45,106.83 X3.A31 | v29.37,156.99 29.69,156.67 v74.14,156.67 | v74.14,149.53 74.45,149.21 83.98,149.21 84.45,148.74 93.5,148.74 94.14,149.37 98.11,149.37 v98.42,149.69 | v28.89,107.3 36.51,107.3 36.99,106.83 37.94,106.83 38.58,106.19 38.89,106.19 39.53,105.56 40.48,105.56 40.64,105.72 40.96,105.72 42.07,106.83 44.93,106.83 X2.A31 | v74.61,106.67 74.29,106.35 67.79,106.35 67.31,106.83 65.72,106.83 X1.A31 | v76.2,126.19 v74.61,126.19 | v74.14,147.47 v76.2,147.47
AD19  (via drill 0.3)
  Top 0.254: v13.97,108.1 13.97,113.81 13.65,114.13 13.65,116.03 13.97,116.35 13.97,118.89 14.29,119.21 14.29,123.65 13.97,123.97 13.97,126.19 13.65,126.51 v13.65,129.37 | v23.02,126.83 23.97,125.88 24.92,125.88 25.4,125.4 v25.72,125.4 | v33.02,125.4 33.02,113.81 32.7,113.49 v32.7,108.1 | v48.26,107.62 48.26,110.16 47.94,110.48 47.94,113.81 48.42,114.29 48.42,116.35 48.74,116.67 48.74,147.47 v48.42,147.78 | v44.45,161.44 v44.45,147.78 | v28.57,161.75 28.57,154.29 28.26,153.98 28.26,149.69 27.46,148.9 27.46,140.32 27.62,140.16 27.62,132.54 28.1,132.07 28.1,130.8 27.78,130.48 27.78,125.72 v28.1,125.4 | v85.88,117.15 85.88,124.13 85.09,124.92 85.09,132.54 v85.41,132.86 | v80.8,133.02 81.12,133.34 81.12,145.88 80.8,146.2 80.8,151.44 v80.49,151.75 | v56.99,148.1 v56.99,151.12
  Bottom 0.152: X6.J3-D16 87.36,117.15 v85.88,117.15
  Bottom 0.254: v13.97,108.1 16.67,108.1 X3.B30 | v13.65,129.37 16.03,129.37 16.35,129.69 17.3,129.69 17.94,129.05 18.26,129.05 18.89,128.42 19.84,128.42 20.48,127.78 20.8,127.78 21.43,127.15 22.38,127.15 22.7,126.83 v23.02,126.83 | v33.02,125.4 v28.1,125.4 v25.72,125.4 | v32.7,108.1 37.31,108.1 X2.B30 | v48.26,107.62 48.58,107.3 56.36,107.3 57.15,108.1 57.94,108.1 X1.B30 | v44.45,147.78 v48.42,147.78 49.05,148.42 56.67,148.42 v56.99,148.1 | v44.45,161.44 37.46,161.44 37.15,161.12 31.11,161.12 30.48,161.75 v28.57,161.75 | v85.41,132.86 85.25,132.7 81.12,132.7 v80.8,133.02 | v80.49,151.75 69.37,151.75 68.74,151.12 63.34,151.12 63.02,150.8 57.31,150.8 v56.99,151.12
AD20  (via drill 0.3)
  Top 0.254: v31.75,108.57 32.23,109.05 32.23,113.81 32.54,114.13 32.54,124.77 32.23,125.08 v32.23,129.85 | v35.72,129.85 35.72,131.75 35.88,131.91 v35.88,139.05 | v33.34,139.05 33.65,139.37 33.65,142.39 33.97,142.7 33.97,146.99 33.34,147.63 33.34,152.86 33.02,153.18 33.02,154.77 32.7,155.09 v32.7,157.47 | v74.93,157.47 74.93,156.36 74.61,156.04 74.61,150.48 v75.09,150.01 75.41,149.69 75.41,140.64 75.09,140.32 75.09,127.78 75.41,127.46 v75.41,109.37 | v100.01,150.48 100.01,148.58 99.69,148.26 99.69,118.42 v99.97,118.14
  Bottom 0.152: X6.J3-B16 92.31,118.22 v99.97,118.14
  Bottom 0.254: X2.A29 45.08,109.37 46.04,109.37 46.67,108.73 46.67,106.99 47.78,106.99 47.94,106.83 58.42,106.83 59.05,107.46 59.53,107.46 60.17,108.1 60.96,108.1 61.44,108.57 61.91,108.57 62.71,109.37 65.56,109.37 X1.A29 65.72,109.37 v75.41,109.37 | v31.75,108.57 31.43,108.89 25.88,108.89 25.4,109.37 24.45,109.37 X3.A29 | v35.72,129.85 v32.23,129.85 | v33.34,139.05 v35.88,139.05 | v32.7,157.47 33.02,157.15 73.5,157.15 73.82,157.47 v74.93,157.47 | v75.09,150.01 75.41,149.69 84.3,149.69 84.77,149.21 93.19,149.21 93.82,149.85 97.47,149.85 98.11,150.48 v100.01,150.48
AD21  (via drill 0.3)
  Top 0.254: v99.54,116.99 99.22,117.3 v99.22,161.28 | v27.78,156.99 v27.78,162.71 | v9.05,156.67 9.37,156.36 9.37,152.39 9.68,152.07 9.68,144.29 10,143.97 10,123.02 9.37,122.38 v9.37,109.68
  Bottom 0.152: X6.J3-A16 arc90 93.58,116.99 v99.54,116.99
  Bottom 0.254: X1.B29 60.48,109.37 46.83,109.37 45.56,110.64 44.61,110.64 43.34,109.37 40,109.37 X2.B29 39.85,109.37 26.19,109.37 24.92,110.64 23.97,110.64 22.7,109.37 19.37,109.37 X3.B29 19.21,109.37 16.35,109.37 16.03,109.68 v9.37,109.68 | v99.22,161.28 95.88,161.28 95.25,160.64 60.8,160.64 59.85,161.6 46.2,161.6 45.08,162.71 43.81,162.71 43.5,162.39 36.83,162.39 36.51,162.07 32.38,162.07 31.75,162.71 v27.78,162.71 | v27.78,156.99 27.46,157.31 14.6,157.31 14.29,156.99 10.48,156.99 10.16,156.67 v9.05,156.67
AD22  (via drill 0.3)
  Top 0.254: v47.47,108.57 47.47,108.73 45.56,110.64 44.61,110.64 44.29,110.32 42.86,110.32 42.54,110.64 X2.A28 | v56.51,108.57 56.83,108.57 57.63,109.37 58.42,109.37 59.37,110.32 59.37,112.38 60.17,113.18 61.12,113.18 63.18,111.11 63.18,110.8 X1.A28 | v13.18,112.22 13.18,116.35 13.49,116.67 13.49,119.21 13.81,119.53 13.81,123.34 13.49,123.65 13.49,125.88 13.18,126.19 13.18,128.73 12.86,129.05 12.86,135.56 14.29,136.99 14.29,141.43 13.97,141.75 13.97,148.74 13.65,149.05 v13.65,158.26 | v76.99,158.26 76.99,147.15 76.36,146.51 76.36,140.01 76.04,139.69 76.04,128.42 76.36,128.1 76.36,127.15 76.99,126.51 v76.99,120.32 | v74.14,110.95 74.45,111.27 74.45,120 v74.14,120.32
  Bottom 0.152: X6.J3-C17 88.76,119.95 arc90 88.51,120.2 81.28,120.16
  Bottom 0.254: v47.47,108.57 47.78,108.89 56.2,108.89 v56.51,108.57 | v13.18,112.22 16.03,112.22 16.35,111.91 17.3,111.91 18.57,110.64 21.75,110.64 X3.A28 | v13.65,158.26 33.02,158.26 33.65,157.63 73.18,157.63 73.5,157.94 74.29,157.94 74.61,158.26 v76.99,158.26 | 81.28,120.16 81.12,120 77.31,120 v76.99,120.32 77.15,120 74.45,120 v74.14,120.32 | v74.14,110.95 66.36,110.95 66.04,110.64 63.18,110.64 X1.A28
AD23  (via drill 0.3)
  Top 0.254: v102.55,120.16 102.55,126.51 102.23,126.83 102.23,135.4 101.6,136.04 101.6,146.51 v101.92,146.83 | v97.95,146.83 97.63,147.15 97.63,158.58 97.95,158.9 v97.95,160.01 | v47.47,160.33 47.47,149.85 47.15,149.53 47.15,139.69 47.31,139.53 47.31,134.29 v46.99,133.97 | v53.97,133.81 54.29,133.5 54.29,126.19 53.97,125.88 v53.97,111.91
  Bottom 0.152: X6.J3-B17 | X6.J3-B17 91.28,119.21 92.39,120.2 101.6,120.16
  Bottom 0.254: X3.B27 19.37,111.91 22.7,111.91 23.97,113.18 24.92,113.18 26.19,111.91 39.85,111.91 X2.B27 40,111.91 43.34,111.91 44.61,113.18 45.56,113.18 46.83,111.91 v53.97,111.91 60.48,111.91 X1.B27 | v102.55,120.16 101.6,120.16 | v101.92,146.83 101.76,146.67 98.11,146.67 v97.95,146.83 | v97.95,160.01 96.84,160.01 96.52,159.69 60.17,159.69 59.21,160.64 54.77,160.64 54.13,160.01 47.78,160.01 v47.47,160.33 | v46.99,133.97 47.31,134.29 53.5,134.29 v53.97,133.81
AD24  (via drill 0.3)
  Top 0.254: v26.03,120.8 26.03,120.48 25.24,120.48 24.92,120.8 23.97,120.8 23.18,120 23.18,116.51 24.45,115.24 24.45,114.61 X3.A25 | v35.08,120.32 35.08,128.26 34.29,129.05 34.29,136.35 34.61,136.67 34.61,141.75 34.92,142.07 34.92,147.63 34.29,148.26 34.29,153.34 36.67,155.72 v36.67,155.88 | v77.79,155.88 77.47,155.56 77.47,150.48 | 77.47,150.48 77.47,146.83 76.83,146.2 76.83,139.69 76.52,139.37 76.52,128.73 76.83,128.42 76.83,127.46 77.47,126.83 77.47,120.96 77.79,120.64 v77.79,118.26 | v69.53,114.76 v69.53,117.62 | v52.07,112.86 52.07,110.48 52.39,110.16 52.39,100.32 v52.07,100 | v53.82,100 54.13,99.68 54.13,90.79 53.34,89.92 v53.34,82.54 | v58.74,83.01 58.74,81.27 59.37,80.63 59.37,78.41 60.17,77.62 60.96,77.62 61.44,78.09 61.91,78.09 62.71,78.89 63.5,78.89 64.77,80.16 64.77,80.95 v65.09,81.27 | v72.55,81.11 72.55,84.76 73.34,85.55 73.34,86.19 73.02,86.51 73.02,102.22 73.34,102.54 v73.34,103.97 | v79.53,103.97 79.85,104.29 79.85,117.62 v79.37,118.1 | v100.96,123.18 100.65,123.5 100.65,129.37 101.28,130 101.28,130.64 100.17,131.75 100.17,147.94 100.49,148.26 100.49,149.85 100.81,150.17 v100.81,151.28 | 77.47,150.48 v77.79,150.48
  Bottom 0.152: X6.J3-A19 arc90 93.39,123.18 100.17,123.18
  Bottom 0.254: v26.03,120.8 26.83,120 34.77,120 v35.08,120.32 | v36.67,155.88 36.99,156.2 73.5,156.2 73.82,155.88 v77.79,155.88 | v69.53,117.62 71.12,117.62 72.07,118.57 77.47,118.57 v77.79,118.26 79.22,118.26 v79.37,118.1 | v69.53,114.76 69.37,114.61 67.47,114.61 67.31,114.45 65.72,114.45 X1.A25 | v52.07,112.86 48.58,112.86 47.47,113.97 46.51,113.97 46.04,114.45 45.08,114.45 X2.A25 | v53.82,100 v52.07,100 | v53.34,82.54 53.34,82.22 55.88,82.22 56.67,83.01 v58.74,83.01 | v65.09,81.27 65.72,81.27 69.85,81.11 v72.55,81.11 | v79.53,103.97 v73.34,103.97 | v100.96,123.18 100.17,123.18 | v100.81,151.28 99.69,151.28 99.38,150.96 97.79,150.96 97.15,150.32 93.5,150.32 92.87,149.69 86.52,149.69 86.2,150.01 84.77,150.01 84.61,150.17 78.1,150.17 v77.79,150.48
AD25  (via drill 0.3)
  Top 0.254: v62.07,114.76 61.12,115.72 60.17,115.72 59.85,115.4 58.42,115.4 58.1,115.72 X1.B24 | v78.58,126.19 v78.58,116.35 | v27.3,116.19 27.3,123.18 v27.62,123.5 | v25.72,123.65 25.24,123.65 24.92,123.34 23.97,123.34 v23.02,124.29 | v14.45,126.83 14.45,124.29 14.76,123.97 14.76,118.89 14.45,118.57 v14.45,115.72 | v49.69,115.72 49.69,153.98 49.53,154.13 49.53,155.09 49.21,155.4 49.21,162.23 49.53,162.55 v49.53,166.36 | v26.19,166.36 26.19,165.25 26.51,164.93 26.51,162.07 26.83,161.75 26.83,157.94 26.51,157.63 26.51,152.86 v26.19,152.55 | v7.62,152.23 7.94,151.91 7.94,151.44 8.25,151.12 8.25,143.34 8.57,143.02 8.57,127.15 v8.25,126.83
  Bottom 0.152: X6.J3-C20 89.36,125.94 arc90 89.11,126.19 81.44,126.19
  Bottom 0.254: v62.07,114.76 62.39,114.76 62.71,114.45 63.5,114.45 64.13,115.08 64.61,115.08 65.25,115.72 66.04,115.72 66.67,116.35 v78.58,116.35 | 81.44,126.19 v78.58,126.19 | v27.3,116.19 27.62,116.51 34.92,116.51 35.72,115.72 37.31,115.72 X2.B24 | v27.62,123.5 27.46,123.65 v25.72,123.65 | v23.02,124.29 22.7,124.29 22.38,124.61 21.43,124.61 20.8,125.24 20.48,125.24 19.84,125.88 18.89,125.88 18.26,126.51 17.94,126.51 17.3,127.15 16.35,127.15 16.03,126.83 v14.45,126.83 v8.25,126.83 | v14.45,115.72 16.67,115.72 X3.B24 | v49.69,115.72 57.94,115.72 X1.B24 | v49.53,166.36 49.21,166.04 27.62,166.04 27.3,166.36 v26.19,166.36 | v26.19,152.55 25.88,152.86 13.33,152.86 13.02,152.55 11.27,152.55 10.95,152.23 v7.62,152.23
AD26  (via drill 0.3)
  Top 0.254: v101.76,126.19 101.76,130.96 100.65,132.07 100.65,147.63 100.96,147.94 100.96,148.58 v101.28,148.9 | v72.55,145.56 v72.55,149.05 | v78.1,145.56 77.79,145.56 77.79,139.05 77.47,138.74 77.47,130.32 v77.79,130 | v72.39,117.15 v72.39,130
  Bottom 0.152: X6.J3-B20 91.36,126.19 101.6,126.19
  Bottom 0.254: 43.81,115.72 43.81,114.61 43.18,114.61 43.02,114.45 41.75,114.45 40.48,115.72 39.21,115.72 37.94,114.45 27.94,114.45 25.4,116.99 24.45,116.99 X3.A23 | 43.81,115.72 43.81,116.35 44.45,116.99 44.93,116.99 X2.A23 | 43.81,115.72 45.56,115.72 46.83,114.45 58.58,114.45 59.85,115.72 60.96,115.72 62.23,116.99 65.56,116.99 X1.A23 65.72,116.99 67.31,116.99 67.47,116.83 69.85,116.83 70.17,117.15 v72.39,117.15 | v101.76,126.19 101.6,126.19 | v101.28,148.9 94.46,148.9 93.82,148.26 84.14,148.26 83.66,148.74 72.87,148.74 v72.55,149.05 | v78.1,145.56 v72.55,145.56 | v72.39,130 v77.79,130
AD27  (via drill 0.3)
  Top 0.254: v81.76,127.31 81.76,131.75 82.07,132.07 82.07,139.21 82.39,139.53 82.39,143.97 82.07,144.29 82.07,146.51 81.76,146.83 81.76,153.98 v81.44,154.29 | v55.09,159.85 v55.09,154.93 | v30.16,153.34 v30.16,160.96 | v10.64,153.02 10.64,144.93 10.95,144.61 10.95,120.16 v10.64,119.84
  Bottom 0.152: X6.J3-D21 87.36,127.31 v81.76,127.31
  Bottom 0.254: X1.B23 60.48,116.99 46.83,116.99 45.56,118.26 44.61,118.26 43.34,116.99 40,116.99 X2.B23 39.85,116.99 26.19,116.99 24.92,118.26 23.97,118.26 22.7,116.99 19.37,116.99 X3.B23 19.21,116.99 18.41,116.99 18.41,118.42 17.3,119.53 16.35,119.53 16.03,119.84 v10.64,119.84 | v81.44,154.29 81.12,154.61 77.15,154.61 76.83,154.93 73.18,154.93 72.87,155.25 55.4,155.25 v55.09,154.93 | v55.09,159.85 55.09,159.53 39.85,159.53 38.42,160.96 37.78,160.96 37.46,160.64 30.48,160.64 v30.16,160.96 | v30.16,153.34 13.02,153.34 12.7,153.02 v10.64,153.02
AD28  (via drill 0.3)
  Top 0.254: v44.13,123.34 44.13,122.86 43.81,122.54 43.81,120.32 42.54,119.05 42.54,118.42 X2.A22 | v46.67,126.35 v46.67,123.34 | v56.51,126.35 56.83,126.35 57.63,127.15 58.42,127.15 59.37,128.1 59.37,130.16 60.17,130.96 61.12,130.96 v62.07,130 | v16.03,116.99 17.3,116.99 17.62,116.67 17.94,116.67 18.89,115.72 19.84,115.72 21.91,117.78 21.91,118.26 X3.A22 | v12.7,116.99 13.02,116.99 13.02,125.56 12.7,125.88 12.7,128.42 12.38,128.73 12.38,135.88 13.81,137.31 13.81,141.12 13.49,141.43 13.49,148.42 13.18,148.74 13.18,157.63 12.86,157.94 v12.86,159.06 | v67.47,158.42 67.47,148.58 68.42,147.63 68.42,133.5 68.1,133.18 68.1,128.26 v67.79,127.94 | v70.17,127.94 v70.17,118.42
  Bottom 0.152: X6.J3-C21 88.57,128 arc90 88.27,128.22 81.28,128.26
  Bottom 0.254: v46.67,123.34 v44.13,123.34 | v46.67,126.35 46.99,126.67 56.2,126.67 v56.51,126.35 | v62.07,130 62.39,130 62.71,129.69 63.66,129.69 64.29,129.05 64.61,129.05 65.25,128.42 66.2,128.42 66.99,127.62 67.79,127.62 | 70.17,127.62 73.98,127.62 74.61,128.26 81.28,128.26 | 70.17,127.62 67.79,127.62 | v12.7,116.99 v16.03,116.99 | v12.86,159.06 13.97,159.06 14.29,158.74 33.34,158.74 33.97,158.1 67.15,158.1 v67.47,158.42 | 67.79,127.62 v67.79,127.94 | v70.17,118.42 66.2,118.42 66.04,118.26 63.18,118.26 X1.A22 | 70.17,127.62 v70.17,127.94
AD29  (via drill 0.3)
  Top 0.254: v103.03,127.15 102.71,127.15 102.71,135.72 102.08,136.35 102.08,145.88 102.71,146.51 v102.71,147.94 | v96.36,147.94 96.68,148.26 96.68,158.58 96.2,159.06 v96.2,160.48 | v31.43,157.47 v31.43,161.91 | v9.84,157.47 9.84,152.71 10.16,152.39 10.16,144.61 10.48,144.29 10.48,122.38 v10.16,122.07 | v17.94,121.91 18.1,121.75 18.1,121.59 19.37,120.32 19.37,119.69 X3.B21
  Bottom 0.152: X6.J3-A21 arc90 93.42,127.15 100.17,127.15
  Bottom 0.254: X3.B21 19.37,119.53 22.7,119.53 23.97,120.8 24.92,120.8 26.19,119.53 39.85,119.53 X2.B21 40,119.53 43.34,119.53 44.61,120.8 45.56,120.8 46.83,119.53 60.48,119.53 X1.B21 | v103.03,127.15 100.17,127.15 | v96.36,147.94 v102.71,147.94 | v96.2,160.48 96.2,160.17 60.48,160.17 59.53,161.12 45.88,161.12 44.77,162.23 44.13,162.23 43.81,161.91 37.15,161.91 36.83,161.6 31.75,161.6 v31.43,161.91 | v31.43,157.47 31.11,157.79 14.29,157.79 13.97,157.47 v9.84,157.47 | v10.16,122.07 17.3,122.07 17.46,121.91 v17.94,121.91
AD30  (via drill 0.3)
  Top 0.254: v39.05,120.96 39.05,121.27 38.73,121.59 38.73,123.81 37.94,124.61 36.99,124.61 35.88,125.72 v35.88,126.35 | 29.37,122.86 29.37,107.94 29.84,107.46 29.84,82.22 29.21,81.59 29.21,71.27 v31.43,69.04 | 29.37,122.86 v29.37,126.35 | v38.42,68.57 39.05,67.93 v39.05,54.44 | v82.23,74.28 v82.23,54.44 | v100.81,74.28 100.81,78.89 100.49,79.2 100.49,82.7 99.85,83.33 99.85,87.78 100.17,88.09 100.17,90 99.85,90.32 99.85,96.98 100.17,97.3 100.17,99.21 99.06,100.32 99.06,108.89 99.38,109.21 99.38,110.32 99.69,110.64 99.69,113.65 100.81,114.76 100.81,118.42 100.17,119.05 100.17,129.85 v100.45,130.44 | 29.37,122.86 v29.69,122.86 | v66.83,120.48 66.52,120.48 66.2,120.8 65.25,120.8 64.45,121.59 63.34,121.59 63.18,121.43 63.18,120.96 X1.A20 | v71.12,118.73 v71.12,120.48 | v80.33,118.57 80.33,101.91 80.01,101.59 80.01,91.43 80.33,91.11 80.33,90.48 80.01,90.16 80.01,88.57 79.69,88.25 79.69,82.7 80.01,82.38 80.01,77.93 80.33,77.62 v80.33,74.28
  Bottom 0.152: X6.J3-B22 92.23,130.2 98.11,130.2 98.11,130.64 v100.45,130.44
  Bottom 0.254: v39.05,120.96 39.21,120.8 42.39,120.8 X2.A20 | v35.88,126.35 35.56,126.67 29.69,126.67 v29.37,126.35 | v31.43,69.04 36.67,69.04 36.99,68.73 37.94,68.73 38.1,68.57 v38.42,68.57 | v82.23,54.44 v39.05,54.44 | v100.81,74.28 98.11,74.28 97.79,74.6 82.55,74.6 v82.23,74.28 v80.33,74.28 | v29.69,122.86 29.37,122.54 25.72,122.54 24.92,123.34 23.97,123.34 23.18,122.54 23.18,122.07 22.7,121.59 22.54,121.59 21.91,120.96 X3.A20 | v71.12,120.48 v66.83,120.48 | v71.12,118.73 71.44,119.05 79.37,119.05 79.69,118.73 80.17,118.73 v80.33,118.57
AD31  (via drill 0.3)
  Top 0.254: v62.07,119.84 61.12,120.8 60.17,120.8 59.85,120.48 58.42,120.48 58.1,120.8 X1.B20 | v70.96,121.43 70.64,121.75 70.64,127.31 70.96,127.62 v70.96,128.73 | v12.22,120.8 11.91,121.11 11.91,144.61 12.22,144.93 v12.22,153.82 | v53.97,151.91 v53.97,153.82 | v78.58,152.55 78.58,150.17 77.95,149.53 77.95,146.51 77.31,145.88 77.31,139.37 76.99,139.05 76.99,129.37 v77.31,129.05 | v46.67,121.27 46.67,116.83 45.56,115.72 44.61,115.72 44.29,115.4 43.97,115.4 43.02,114.45 42.07,114.45 41.75,114.76 41.43,114.76 40.48,115.72 39.53,115.72 38.73,116.51 38.73,118.73 37.46,120 37.46,120.8 X2.B20
  Bottom 0.152: X6.J3-D22 87.36,129.05 80.01,129.05
  Bottom 0.254: v62.07,119.84 62.39,119.84 62.71,119.53 63.5,119.53 64.13,120.16 64.61,120.16 65.25,120.8 66.04,120.8 66.52,121.27 70.8,121.27 v70.96,121.43 | 77.31,128.73 79.69,128.73 80.01,129.05 | 77.31,128.73 v70.96,128.73 | v12.22,120.8 16.67,120.8 X3.B20 | v12.22,153.82 29.53,153.82 29.84,154.13 34.29,154.13 34.61,153.82 35.4,153.82 35.72,153.5 36.51,153.5 36.83,153.18 47.31,153.18 47.62,153.5 53.66,153.5 v53.97,153.82 | v53.97,151.91 57.31,151.91 57.94,151.28 62.71,151.28 63.02,151.59 68.42,151.59 69.06,152.23 78.26,152.23 v78.58,152.55 | 77.31,128.73 v77.31,129.05 | v46.67,121.27 46.99,121.59 56.04,121.59 56.83,120.8 57.94,120.8 X1.B20
C/BE0#  (via drill 0.3, 0.7)
  Top 0.152: X6.J3-A4 92.4,94.17 92.35,94.17 92.35,95.99 92.39,96.19 90.37,96.23 90.37,102.22 85.57,102.22 v85.57,103.65 | 59.37,81.27 59.37,83.65
  Top 0.203: v66.83,95.4 66.83,85.24 64.45,85.24 64.45,81.59 arc-90 64.29,81.43 X1.A52 60.46,80.18 59.37,81.27 | v82.07,103.65 81.76,103.49 81.76,99.84 80.96,98.73 v80.96,96.98 | 59.37,83.65 59.05,83.97 57.47,83.97 57.47,84.05 56.83,84.68 56.83,86.11 v56.91,86.19 | v52.63,85.71 52.63,80.87 v53.1,80.32
  Bottom 0.203: X3.A52 23.3,81.59 24.61,81.59 25.08,82.06 27.3,82.06 27.78,81.59 34.29,81.59 35.16,82.46 38.5,82.46 38.73,82.22 38.73,81.43 39.98,80.18 X2.A52 43.28,80.95 46.04,80.95 46.67,80.32 v53.1,80.32 | v66.83,95.4 78.42,95.24 78.42,96.98 v80.96,96.98 | v85.57,103.65 v82.07,103.65 | v56.91,86.19 56.75,86.19 56.42,86.08 | 56.42,86.08 56.28,86.03 | v52.63,85.71 52.94,86.03 56.37,86.03 56.42,86.08
C/BE1#  (via drill 0.3)
  Top 0.152: 54.69,85.79 54.69,83.49
  Top 0.203: 54.69,85.79 54.21,86.27 v54.21,89.84 54.45,89.84
  Top 0.254: v12.86,90.32 12.86,89.05 13.97,87.94 13.97,78.25 13.65,77.93 v13.65,65.87 | v27.62,89.84 27.62,84.92 27.3,84.6 27.3,66.19 v27.62,65.87 v27.62,62.22 | 54.69,83.49 54.69,82.93 55.88,81.74 55.88,63.65 55.4,63.17 v55.4,62.54 v55.4,57.77 | v105.41,102.22 105.41,98.89 104.77,98.25 104.77,89.21 104.14,88.57 104.14,76.82 104.46,76.51 104.46,73.33 105.09,72.7 v105.09,69.04 | v80.33,68.89 80.33,65.08 80.17,64.92 v80.17,63.33 | v74.45,63.33 74.45,59.84 73.98,59.36 v73.98,57.14
  Bottom 0.152: X6.J3-B8 91.36,102.22 101.6,102.22
  Bottom 0.203: 57.94,90.32 57.94,90.16 57.63,89.84 v54.21,89.84
  Bottom 0.254: v12.86,90.32 16.67,90.32 X3.B44 | v27.62,65.87 v13.65,65.87 | v27.62,89.84 27.94,89.52 35.4,89.52 36.19,90.32 37.31,90.32 X2.B44 | v55.4,62.54 55.09,62.85 48.1,62.85 47.78,63.17 42.54,63.17 41.91,62.54 35.72,62.54 35.4,62.22 v27.62,62.22 | 57.94,90.32 X1.B44 | v105.41,102.22 101.6,102.22 | v105.09,69.04 101.28,69.04 100.96,69.36 92.71,69.36 91.6,68.25 90.96,68.25 90.33,68.89 v80.33,68.89 | v80.17,63.33 79.85,63.01 75.09,63.01 74.77,63.33 v74.45,63.33 | v73.98,57.14 64.77,57.14 63.82,58.09 55.72,58.09 v55.4,57.77
C/BE2#  (via drill 0.3)
  Top 0.254: v82.23,113.18 82.23,124.45 82.55,124.77 82.55,130.48 82.23,130.8 82.23,131.43 82.55,131.75 82.55,138.89 82.87,139.21 82.87,144.29 82.55,144.61 82.55,146.83 82.23,147.15 v82.23,155.09 | v38.1,160.17 v38.1,155.4 | v16.99,161.12 16.99,160.01 17.3,159.69 17.3,145.56 v16.99,145.24 | v11.43,107.3 v11.43,145.24 | v17.94,106.51 19.37,105.08 19.37,104.45 X3.B33
  Bottom 0.152: X6.J3-D14 87.36,113.18 v82.23,113.18
  Bottom 0.254: X3.B33 19.37,104.29 22.7,104.29 23.97,105.56 24.92,105.56 26.19,104.29 39.85,104.29 X2.B33 40,104.29 43.34,104.29 44.61,105.56 45.56,105.56 46.83,104.29 60.48,104.29 X1.B33 | v82.23,155.09 77.47,155.09 77.15,155.4 73.5,155.4 73.18,155.72 38.42,155.72 v38.1,155.4 | v38.1,160.17 25.4,160.17 24.76,160.8 18.41,160.8 18.1,161.12 v16.99,161.12 | v11.43,145.24 v16.99,145.24 | v11.43,107.3 15.87,107.3 16.35,106.83 17.3,106.83 17.62,106.51 v17.94,106.51
C/BE3#  (via drill 0.3)
  Top 0.254: v8.1,113.18 8.41,113.49 8.41,123.02 9.05,123.65 9.05,143.34 8.73,143.66 8.73,151.44 8.41,151.75 8.41,154.29 v8.1,154.61 | v48.89,113.65 48.89,116.03 49.21,116.35 49.21,153.66 48.89,153.98 48.89,154.61 v48.74,154.77 v48.74,162.87 | v33.5,112.86 33.5,105.56 v33.34,105.4 | v31.11,105.4 30.8,105.08 30.8,81.59 30.16,80.95 30.16,73.01 32.23,70.95 32.23,68.09 31.27,67.14 v31.27,66.5 | v23.18,66.66 23.02,66.5 v23.02,63.65 | v2.06,63.01 1.27,63.81 1.27,112.38 v2.06,113.18 | v107.16,124.29 107.16,134.45 106.52,135.08 106.52,143.5 105.89,144.13 105.89,155.56 106.52,156.2 v106.52,162.87
  Bottom 0.152: X6.J3-B19 92.31,124.21 101.52,124.21
  Bottom 0.254: v8.1,154.61 12.54,154.61 12.86,154.29 26.35,154.29 27.46,155.4 28.1,155.4 28.42,155.09 34.92,155.09 35.24,154.77 36.04,154.77 36.35,154.45 37.15,154.45 37.46,154.13 46.67,154.13 46.99,154.45 48.42,154.45 v48.74,154.77 | v48.89,113.65 49.21,113.97 56.04,113.97 56.83,113.18 57.94,113.18 X1.B26 | X3.B26 16.67,113.18 v8.1,113.18 v2.06,113.18 | v33.5,112.86 34.61,112.86 34.92,113.18 37.31,113.18 X2.B26 | v31.11,105.4 v33.34,105.4 | v31.27,66.5 29.21,66.5 28.89,66.82 27.46,66.82 26.99,66.35 23.49,66.35 v23.18,66.66 | v23.02,63.65 22.7,63.96 16.51,63.96 15.87,63.33 12.22,63.33 11.91,63.01 v2.06,63.01 | v107.16,124.29 101.52,124.21 | v106.52,162.87 103.98,162.87 103.66,162.55 98.58,162.55 98.27,162.23 95.25,162.23 94.61,161.6 61.44,161.6 60.48,162.55 49.05,162.55 v48.74,162.87
CLK1  (via drill 0.3)
  Top 0.254: v54.77,125.56 54.77,134.13 55.56,134.93 55.56,135.4 55.88,135.72 55.88,137.62 55.72,137.78 55.72,143.34 55.24,143.82 55.24,152.39 55.56,152.71 v55.56,153.82 | v79.69,153.18 79.69,151.44 80.33,150.8 80.33,145.88 80.64,145.56 80.64,137.47 v80.33,137.15
  Bottom 0.152: X6.J3-D26 87.36,137.15 v80.33,137.15 80.01,137.15
  Bottom 0.254: v54.77,125.56 56.83,125.56 57.15,125.88 57.94,125.88 X1.B16 | v55.56,153.82 56.67,153.82 56.83,153.66 57.47,153.66 58.1,154.29 72.23,154.29 72.55,153.98 76.2,153.98 76.52,153.66 79.22,153.66 v79.69,153.18
CLK2  (via drill 0.3)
